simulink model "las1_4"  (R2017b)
settings: Solver=ode45  StartTime=0.0  StopTime=300  MaxStep=1  RelTol=1e-3  AbsTol=1e-3

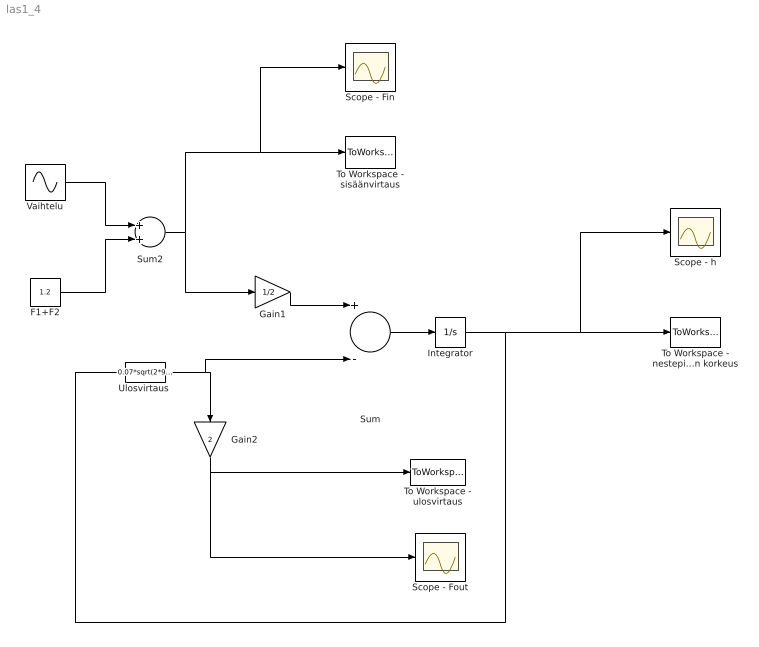
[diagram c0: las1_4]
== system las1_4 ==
  F1+F2 : Constant  Value=1.2
  Gain1 : Gain  Gain=1/2
  Gain2 : Gain  Gain=2
  Integrator : Integrator  InitialCondition=10
  Scope - Fin : Scope
  Scope - Fout : Scope
  Scope - h : Scope
  Sum : Sum  Inputs=+-
  Sum2 : Sum
  To Workspace - ulosvirtaus : ToWorkspace  VariableName=Fout
  To Workspace - nestepinnan korkeus : ToWorkspace  VariableName=h
  To Workspace - sisäänvirtaus : ToWorkspace  VariableName=Fin
  "Ulosvirtaus " : Fcn  Expr=0.07*sqrt(2*9.81*u)/2
  Vaihtelu : Sin  Amplitude=0.5  Frequency=0.5  SampleTime=0.1
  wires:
  Sum2/1 -> To Workspace - sisäänvirtaus/1, Scope - Fin/1, Gain1/1
  Sum/1 -> Integrator/1
  "Ulosvirtaus "/1 -> Sum/2, Gain2/1
  F1+F2/1 -> Sum2/2
  Integrator/1 -> "Ulosvirtaus "/1, To Workspace - nestepinnan korkeus/1, Scope - h/1
  Vaihtelu/1 -> Sum2/1
  Gain1/1 -> Sum/1
  Gain2/1 -> To Workspace - ulosvirtaus/1, Scope - Fout/1
